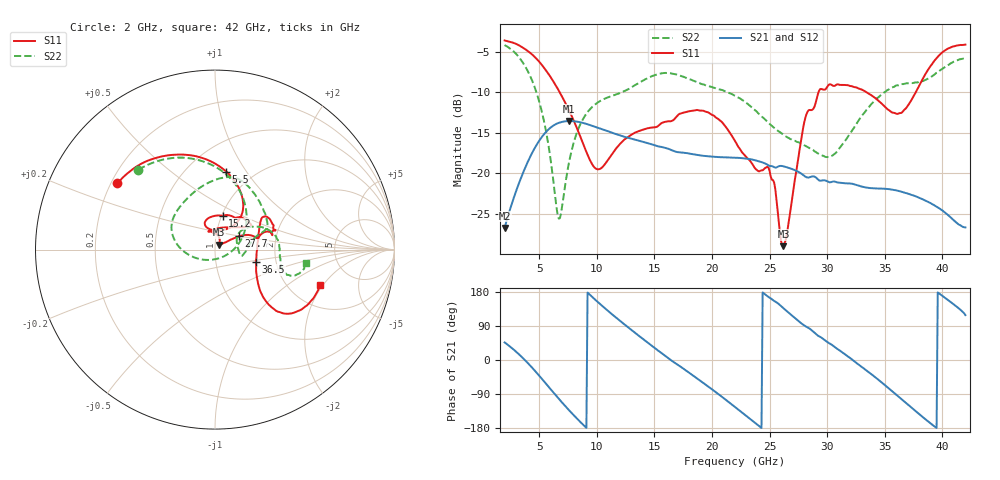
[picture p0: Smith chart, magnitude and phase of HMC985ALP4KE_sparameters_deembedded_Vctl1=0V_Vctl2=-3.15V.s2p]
!s2p File: Measurements: S11, S21, S12, S22
# GHz S dB R 50.0
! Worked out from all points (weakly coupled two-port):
!   401 points, 2 GHz to 42 GHz, reference 50 ohm
!   highest |S21| = -13.55 dB at 7.6 GHz (marker M1); lowest = -26.7 dB at 2 GHz (marker M2)
!   lowest |S11| = -28.9 dB at 26.2 GHz (marker M3), VSWR 1.07, Z = 52.3 + j2.87 ohm
!   |S11| at or under -10 dB: 6.776 GHz to 29.25 GHz (22.48 GHz wide, 125 % of centre); 33.4 GHz to 37.7 GHz (4.294 GHz wide, 12.1 % of centre)
!   |S22| runs from -25.5 to -4.2 dB; largest |S21 - S12| = 0.0006
!   S11 on the Smith chart (normalised r, x): 2 GHz: 0.22, +0.29; 5.5 GHz: 0.76, +0.81; 15.2 GHz: 1.01, +0.40; 27.7 GHz: 1.29, +0.20; 36.5 GHz: 1.57, -0.22; 42 GHz: 2.93, -1.90
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2  -3.64 145.9  -26.70 46.4  -26.69 46.5  -4.21 133.8
3.6  -4.54 118.4  -19.92 4.7  -19.94 4.7  -6.41 93.6
5.5  -7.15 81.8  -15.04 -59.1  -15.06 -59.1  -14.11 32.4
6.7  -9.81 61.7  -13.78 -102.1  -13.77 -102.1  -25.55 -68.8
7.6  -12.26 52.5  -13.55 -132.8  -13.56 -132.8  -18.56 -157.0
8.7  -15.93 53.6  -13.74 -167.3  -13.74 -167.3  -13.58 173.2
10.2  -19.48 89.0  -14.43 150.0  -14.40 150.0  -11.16 151.1
12.5  -15.73 110.1  -15.53 91.5  -15.50 91.6  -9.80 118.8
15.2  -14.28 77.1  -16.61 27.6  -16.61 27.6  -7.83 82.1
15.4  -14.07 74.7  -16.69 23.3  -16.71 23.2  -7.74 80.1
19.2  -12.28 33.6  -17.82 -59.4  -17.82 -59.4  -9.04 41.7
22  -16.00 51.9  -18.06 -124.0  -18.08 -124.0  -10.44 21.4
24.9  -19.25 104.0  -19.00 166.5  -18.98 166.5  -13.75 11.5
26.2  -28.94 50.1  -19.12 136.8  -19.13 136.8  -15.23 -2.3
27.7  -16.26 28.9  -19.97 98.2  -20.00 98.2  -16.30 -13.3
28.7  -12.17 12.9  -20.36 77.4  -20.35 77.4  -17.05 -10.2
31  -9.06 23.2  -21.12 27.0  -21.09 26.9  -17.02 28.9
33.3  -9.91 34.2  -21.71 -25.1  -21.70 -25.0  -12.41 31.8
35.4  -12.25 11.8  -21.93 -76.1  -21.93 -76.2  -9.62 17.2
36.5  -12.50 -16.5  -22.27 -104.5  -22.27 -104.5  -9.00 8.1
39.5  -5.84 -43.5  -24.09 -179.4  -24.06 -179.4  -7.62 -18.6
42  -4.15 -18.8  -26.64 118.4  -26.65 118.5  -5.85 -8.4
